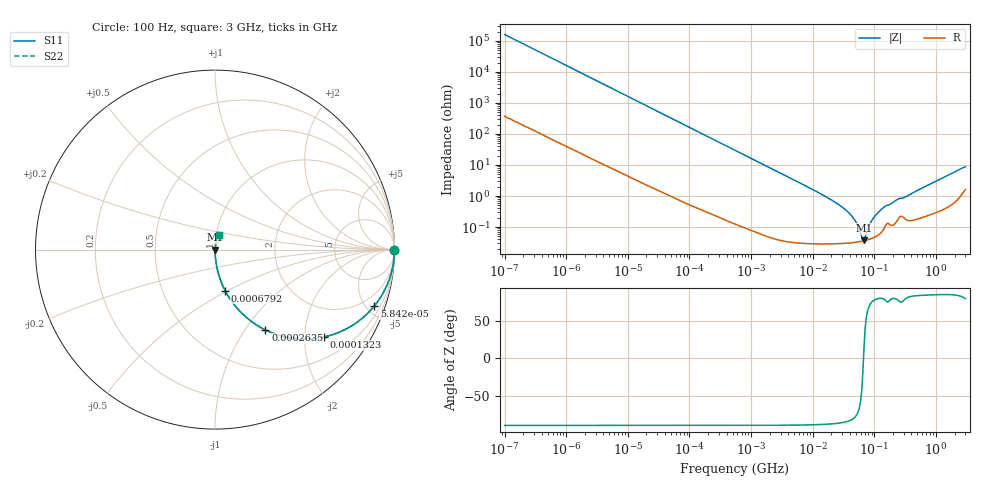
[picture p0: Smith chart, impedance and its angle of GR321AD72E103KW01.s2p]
!Murata Part Number: GR321AD72E103KW01
!These Parameters are Measured in Series Mode Connection
!Data Generated on Jan 08, 2026
!  o--ll--o
!Port1  Port2
!  o------o
!Operation Temp=25[degC], DC Bias Voltage=0[V]
!Freq. Start=100[Hz] Stop=3[GHz] 401[Steps]
# Hz S RI R 50
!Freq.(Hz) S11(Real) S11(Imag) S21(Real) S21(Imag) S12(Real) S12(Imag) S22(Real) S22(Imag)
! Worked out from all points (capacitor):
!   401 points, 100 Hz to 3 GHz, reference 50 ohm
!   read as one part in series: C = 9.8 nF near 109 Hz
!   lowest |Z| = 37.2 mohm at 67.94 MHz (marker M1)
!   series resonance near 66.71 MHz, so ESL is about 580 pH
!   S11 on the Smith chart (normalised r, x): 100 Hz: open; 58.42 kHz: 1.02, -5.62; 132.3 kHz: 1.01, -2.48; 263.5 kHz: 1.00, -1.25; 679.2 kHz: 1.00, -0.49; 3 GHz: 1.03, +0.17
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100  1 -0.000616  1.8e-06 0.000616  1.8e-06 0.000616  1 -0.000616
1788  0.9999 -0.011  0.000148 0.011  0.000148 0.011  0.9999 -0.011
10003  0.9961 -0.0609  0.00389 0.0609  0.00389 0.0609  0.9961 -0.0609
31977  0.9628 -0.1877  0.0372 0.1877  0.0372 0.1877  0.9628 -0.1877
58416  0.8868 -0.3154  0.1132 0.3154  0.1132 0.3154  0.8868 -0.3154
132342  0.6062 -0.4869  0.3938 0.4869  0.3938 0.4869  0.6062 -0.4869
263501  0.2813 -0.4478  0.7187 0.4478  0.7187 0.4478  0.2813 -0.4478
547723  0.084 -0.2753  0.916 0.2753  0.916 0.2753  0.084 -0.2753
679242  0.0565 -0.2288  0.9435 0.2288  0.9435 0.2288  0.0565 -0.2288
1992254  0.00728 -0.0823  0.9927 0.0823  0.9927 0.0823  0.00728 -0.0823
9794414  0.000562 -0.0165  0.9994 0.0165  0.9994 0.0165  0.000562 -0.0165
2.316512e7  0.000329 -0.00628  0.9997 0.00628  0.9997 0.00628  0.000329 -0.00628
3.71925e7  0.000312 -0.00307  0.9997 0.00307  0.9997 0.00307  0.000312 -0.00307
4.815176e7  0.000322 -0.00165  0.9997 0.00165  0.9997 0.00165  0.000322 -0.00165
6.234031e7  0.000347 -0.000336  0.9997 0.000336  0.9997 0.000336  0.000347 -0.000336
6.794454e7  0.000361 9.23e-05  0.9996 -9.23e-05  0.9996 -9.23e-05  0.000361 9.23e-05
7.093284e7  0.000368 0.000307  0.9996 -0.000307  0.9996 -0.000307  0.000368 0.000307
8.425944e7  0.000409 0.00118  0.9996 -0.00118  0.9996 -0.00118  0.000409 0.00118
1.000898e8  0.000472 0.00209  0.9995 -0.00209  0.9995 -0.00209  0.000472 0.00209
1.352818e8  0.000756 0.00392  0.9992 -0.00392  0.9992 -0.00392  0.000756 0.00392
1.751444e8  0.00125 0.00509  0.9988 -0.00509  0.9988 -0.00509  0.00125 0.00509
3e9  0.023 0.0827  0.977 -0.0827  0.977 -0.0827  0.023 0.0827
